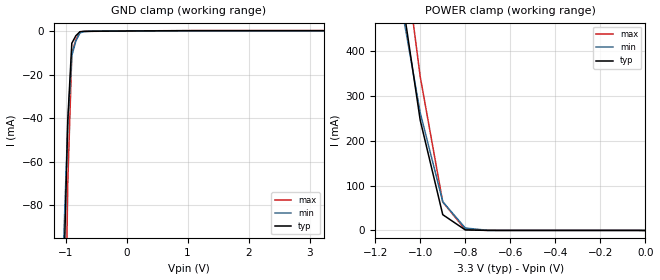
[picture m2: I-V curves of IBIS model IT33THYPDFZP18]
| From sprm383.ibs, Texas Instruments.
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|   Model IT33THYPDFZP18
[Model]   IT33THYPDFZP18
Model_type   Input
Polarity   Non-Inverting
Vinl =  0.8V
Vinh =  2V
C_comp   0.5121187p   0.4653817p   0.5743862p
[Model Spec]
Vinl   0.8V   0.8V   0.8V
Vinh   2V   2V   2V
[Temperature Range]   25   105   0
[Voltage Range]   3.3   3.14   3.47
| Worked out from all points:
|   GND clamp passes 1 mA (typ) near -0.79 V on its own axis
|   POWER clamp passes 1 mA (typ) near -0.78 V on its own axis
[POWER_clamp]
|   voltage   I(typ)   I(min)   I(max)
-3.3V     9.936A     8.589A     10.91A
-1.067V   472.1mA    454mA      602.9mA
-1.033V   359.2mA    358.5mA    473.3mA
-1V       246.3mA    263mA      343.6mA
-900mV    35.33mA    64.33mA    63.64mA
-800mV    1.257mA    5.509mA    1.974mA
-700mV    169.5uA    409.5uA    227.7uA
-11.55fV  0A         0A         0A
[GND_clamp]
|   voltage   I(typ)   I(min)   I(max)
-3.3V     -13.46A    -11.58A    -14.63A
-1.033V   -115.6mA   -96.43mA   -194.3mA
-966.7mV  -41.07mA   -42.98mA   -70.4mA
-900mV    -5.626mA   -11.31mA   -10.56mA
-833.3mV  -2.16mA    -4.573mA   -3.846mA
-766.7mV  -338.9uA   -899.1uA   -392uA
-700mV    -161.6uA   -288.1uA   -200.5uA
-500mV    -104.6uA   -68.65uA   -133.8uA
3.233V    142.6uA    86.74uA    196.8uA
